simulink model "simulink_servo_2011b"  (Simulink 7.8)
settings: Solver=ode4  StartTime=0.0  StopTime=20  FixedStep=1e-2  RelTol=1e-3
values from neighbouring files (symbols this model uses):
  A = [0 1 0 0; -4 -2 4 2; 0 0 0 1; 2 1 -2 -1]    [servo.m]
  B = [0; 2; 0; 0]    [servo.m]
  C = [0 0 1 0]    [servo.m]
  G = Ke(5)    [servo.m]
  K = Ke(1:4)    [servo.m]

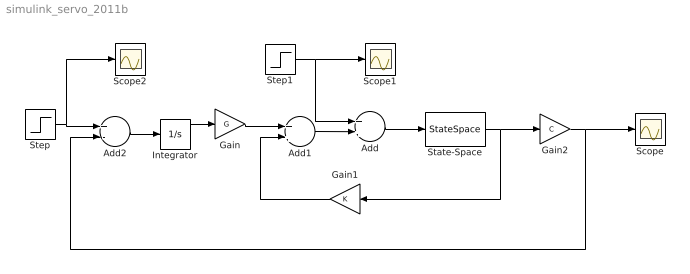
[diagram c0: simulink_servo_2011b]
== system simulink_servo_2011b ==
  Add : Sum
  Add1 : Sum
  Add2 : Sum  Inputs=+-
  Gain : Gain  Gain=G  Multiplication=Matrix(K*u) (u vector)
  Gain1 : Gain  Gain=K  Multiplication=Matrix(K*u) (u vector)
  Gain2 : Gain  Gain=C  Multiplication=Matrix(K*u) (u vector)
  Integrator : Integrator
  Scope : Scope
  Scope1 : Scope
  Scope2 : Scope
  State-Space : StateSpace  A=A  B=B  C=eye(4)  D=zeros(4,1)  X0=zeros(4,1)
  Step : Step  Time=0  SampleTime=0
  Step1 : Step  Time=5  SampleTime=0
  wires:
  Gain/1 -> Add1/1
  Add1/1 -> Add/2
  Add/1 -> State-Space/1
  State-Space/1 -> Gain2/1, Gain1/1
  Gain1/1 -> Add1/2
  Step1/1 -> Add/1, Scope1/1
  Gain2/1 -> Scope/1, Add2/2
  Step/1 -> Scope2/1, Add2/1
  Add2/1 -> Integrator/1
  Integrator/1 -> Gain/1
